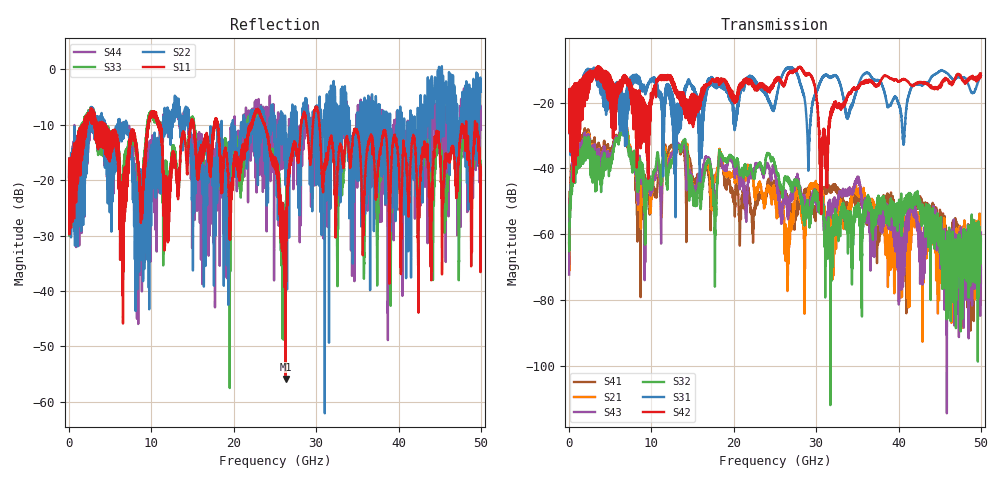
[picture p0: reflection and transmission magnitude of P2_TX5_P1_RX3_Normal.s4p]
!Keysight Technologies,N5225B,MY57041031,A.13.20.10
!Date: Friday, May 31, 2019 11:18:20
!Correction: S11(Full 4 Port(1,2,3,4))
!S12(Full 4 Port(1,2,3,4))
!S13(Full 4 Port(1,2,3,4))
!S14(Full 4 Port(1,2,3,4))
!S21(Full 4 Port(1,2,3,4))
!S22(Full 4 Port(1,2,3,4))
!S23(Full 4 Port(1,2,3,4))
!S24(Full 4 Port(1,2,3,4))
!S31(Full 4 Port(1,2,3,4))
!S32(Full 4 Port(1,2,3,4))
!S33(Full 4 Port(1,2,3,4))
!S34(Full 4 Port(1,2,3,4))
!S41(Full 4 Port(1,2,3,4))
!S42(Full 4 Port(1,2,3,4))
!S43(Full 4 Port(1,2,3,4))
!S44(Full 4 Port(1,2,3,4))
!S4P File: Measurements: <S11,S12,S13,S14>,
!<S21,S22,S23,S24>,
!<S31,S32,S33,S34>,
!<S41,S42,S43,S44>:
# Hz S  dB  R 50.0
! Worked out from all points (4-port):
!   5000 points, 10 MHz to 50 GHz, reference 50 ohm
!   strongest paths, dB at 10 MHz, 12.51 GHz, 25.01 GHz, 37.51 GHz, 50 GHz:
!     S42: -19.5, -14.2, -13.2, -14.5, -11.1
!     S31: -19.5, -17.7, -20.9, -13.1, -11.7
!     S32: -61.0, -37.7, -39.5, -49.2, -61.6
!     S43: -72.3, -35.6, -41.7, -54.6, -59.5
!     S21: -59.4, -35.4, -48.0, -54.0, -70.6
!     S41: -62.7, -33.4, -45.3, -61.2, -74.9
!   lowest |S11| = -55.9 dB at 26.29 GHz (marker M1), VSWR 1.00, Z = 50 - j0.156 ohm
!   |S11| at or under -10 dB: 4.282 GHz to 9.568 GHz (5.286 GHz wide, 76.3 % of centre); 23.74 GHz to 28.18 GHz (4.441 GHz wide, 17.1 % of centre); 30.39 GHz to 47.7 GHz (17.32 GHz wide, 44.3 % of centre)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
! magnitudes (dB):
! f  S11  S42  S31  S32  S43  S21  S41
! 10 MHz  -19.7  -19.5  -19.5  -61.0  -72.3  -59.4  -62.7
! 1.01 GHz  -15.9  -20.0  -18.0  -35.3  -33.1  -32.8  -30.8
! 6.5 GHz  -40.8  -14.9  -19.0  -28.6  -27.8  -28.3  -28.1
! 22.88 GHz  -7.2  -15.7  -14.7  -39.7  -39.2  -46.1  -48.6
! 26.29 GHz  -55.9  -13.1  -9.7  -42.9  -48.2  -57.0  -47.8
! 30.63 GHz  -17.1  -40.2  -13.1  -48.8  -48.3  -45.9  -46.2
! 50 GHz  -19.1  -11.1  -11.7  -61.6  -59.5  -70.6  -74.9
